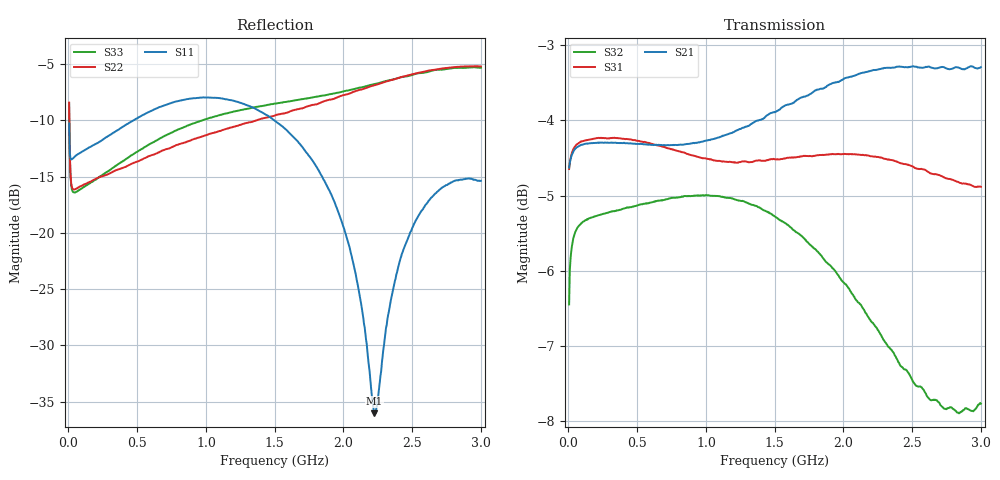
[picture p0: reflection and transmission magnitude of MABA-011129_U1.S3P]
!Agilent Technologies,E5071C,MY46630996,B.13.30
!Date: Tue Aug 16 20:40:59 2022 DD
!Data & Calibration Information:
!MABA-011129-TB soldered onto PT-0028476 with SMA connectors, Port1 (pin1) Port2 (pin4) Port3 (pin3)
!Freq	S11:SOLT3(ON)	S12:SOLT3(ON)	S13:SOLT3(ON)
!	S21:SOLT3(ON)	S22:SOLT3(ON)	S23:SOLT3(ON)
!	S31:SOLT3(ON)	S32:SOLT3(ON)	S33:SOLT3(ON)
!PortZ  Port1:50+j0  Port2:50+j0  Port3:50+j0
!Above PortZ is port z conversion or system Z0 setting when saving the data.
!When reading, reference impedance value at option line is always used.
# Hz S dB R 50
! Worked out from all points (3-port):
!   600 points, 5 MHz to 3 GHz, reference 50 ohm
!   strongest paths, dB at 5 MHz, 755 MHz, 1.505 GHz, 2.255 GHz, 3 GHz:
!     S21: -4.6, -4.3, -3.9, -3.3, -3.3
!     S31: -4.6, -4.4, -4.5, -4.5, -4.9
!     S32: -6.4, -5.0, -5.3, -6.8, -7.8
!   lowest |S11| = -36.0 dB at 2.225 GHz (marker M1), VSWR 1.03, Z = 48.4 + j0.0829 ohm
!   |S11| at or under -10 dB: start of sweep to 473.6 MHz; 1.496 GHz to end of sweep
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5000000  -10.28 61.8  -4.68 -167.0  -4.69 13.0
         -4.63 -167.0  -8.43 92.5  -6.45 30.3
         -4.65 12.9  -6.45 30.2  -8.47 93.2
4.5e7  -13.24 4.3  -4.39 178.3  -4.35 -1.5
       -4.39 178.3  -16.15 23.4  -5.51 3.0
       -4.35 -1.5  -5.51 3.0  -16.42 21.8
6.2e8  -9.06 -100.4  -4.34 126.1  -4.26 -53.9
       -4.33 126.0  -13.06 -53.6  -5.09 -29.0
       -4.32 -53.8  -5.08 -29.1  -11.94 -70.9
1.085e9  -8.01 -152.9  -4.24 86.9  -4.41 -94.3
         -4.23 86.7  -11.00 -79.6  -5.03 -53.7
         -4.54 -93.6  -5.01 -54.0  -9.60 -100.4
1.505e9  -10.08 165.9  -3.92 51.0  -4.50 -130.4
         -3.89 50.7  -9.55 -93.9  -5.30 -77.1
         -4.52 -129.4  -5.28 -77.8  -8.52 -116.9
1.99e9  -19.09 124.6  -3.51 7.7  -4.52 -173.5
        -3.46 7.4  -7.80 -107.4  -6.13 -104.0
        -4.45 -172.9  -6.13 -104.7  -7.46 -131.2
2.225e9  -36.03 176.9  -3.40 -13.9  -4.57 165.0
         -3.33 -14.3  -6.89 -114.9  -6.72 -116.3
         -4.48 165.1  -6.72 -116.6  -6.78 -138.0
2.36e9  -25.09 -113.5  -3.36 -26.4  -4.62 152.4
        -3.30 -26.8  -6.39 -120.0  -7.10 -122.8
        -4.53 152.3  -7.08 -122.9  -6.38 -142.3
2.515e9  -19.17 -117.5  -3.34 -40.8  -4.66 137.8
         -3.29 -41.2  -5.87 -126.1  -7.56 -129.5
         -4.63 137.5  -7.49 -129.3  -5.92 -147.5
3e9  -15.38 -141.2  -3.35 -85.7  -4.84 91.5
     -3.29 -85.4  -5.22 -145.1  -7.97 -147.7
     -4.88 91.3  -7.77 -147.3  -5.34 -162.5
